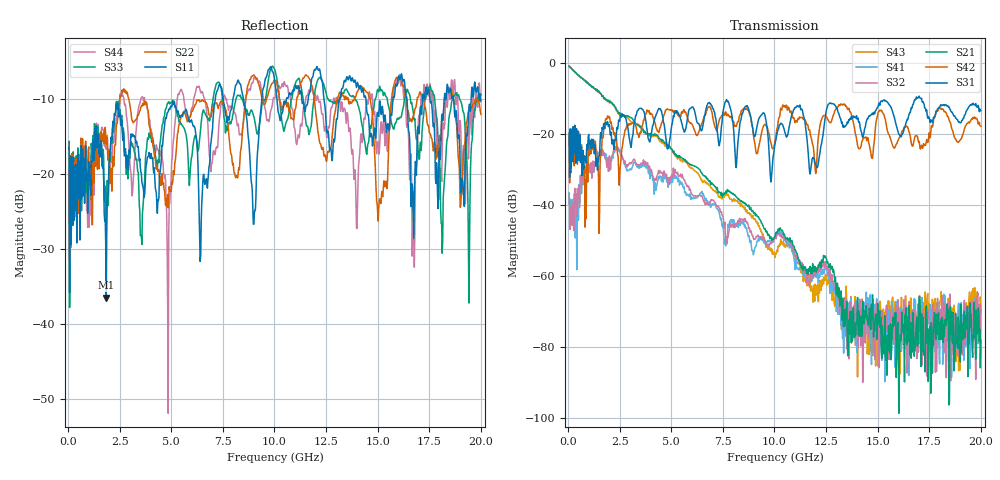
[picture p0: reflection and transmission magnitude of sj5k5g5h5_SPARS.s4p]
! FILE: E:\users\goganessyan\GBX_Backplane\FR408_backplane\1m_OUTBOUND_TRU\sj5k5g5h5_SPARS.s4p
# MHZ S RI R 50.00
! FREQ  S11  S12  S13  S14
!  S21  S22  S23  S24
!  S31  S32  S33  S34
!  S41  S42  S43  S44
!  REAL  IMAG  REAL  IMAG  REAL  IMAG  REAL  IMAG
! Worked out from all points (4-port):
!   799 points, 50 MHz to 20 GHz, reference 50 ohm
!   strongest paths, dB at 50 MHz, 5.025 GHz, 10.03 GHz, 15.03 GHz, 20 GHz:
!     S31: -19.8, -17.6, -22.7, -12.4, -13.6
!     S42: -20.0, -13.5, -22.2, -14.0, -17.9
!     S21: -1.0, -24.3, -49.0, -73.6, -78.1
!     S32: -36.9, -31.5, -49.2, -73.1, -69.5
!     S41: -36.6, -32.3, -48.8, -67.7, -69.8
!     S43: -1.1, -24.6, -54.8, -85.4, -69.4
!   lowest |S11| = -36.5 dB at 1.85 GHz (marker M1), VSWR 1.03, Z = 49.8 + j1.48 ohm
!   |S11| at or under -10 dB: start of sweep to 7.136 GHz; 8.496 GHz to 9.388 GHz (892 MHz wide, 9.98 % of centre); 14.43 GHz to 15.74 GHz (1.317 GHz wide, 8.73 % of centre)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
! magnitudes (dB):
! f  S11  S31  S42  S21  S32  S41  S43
! 50 MHz  -15.8  -19.8  -20.0  -1.0  -36.9  -36.6  -1.1
! 1.85 GHz  -36.5  -17.5  -15.9  -10.4  -27.4  -27.1  -10.4
! 4.85 GHz  -11.7  -23.9  -13.2  -23.3  -33.2  -35.1  -23.8
! 5.425 GHz  -12.5  -15.3  -14.9  -26.8  -31.9  -33.3  -27.4
! 13.43 GHz  -7.7  -17.9  -12.0  -74.1  -68.3  -75.7  -70.8
! 18.12 GHz  -12.1  -12.0  -13.1  -71.7  -65.6  -68.0  -69.4
! 20 GHz  -9.4  -13.6  -17.9  -78.1  -69.5  -69.8  -69.4
